| TEXAS INSTRUMENTS INCORPORATED
| Standard Linear and Logic Group
| IBIS Model of SN74CBT3253C
| Dual 1-Of-4 FET Multiplexer/Demultiplexer
| With -2 V Undershoot-Protection
| This file contains package information for the following:
|  SOIC 16-pin (D) package as [Component] CBT3253C_D
|  SSOP 16-pin (DB) package as [Component] CBT3253C_DB
|  SSOP 16-pin (DBQ) package as [Component] CBT3253C_DBQ
|  TSSOP 16-pin (PW) package as [Component] CBT3253C_PW
|  QFN 16-pin (RGY) package as [Component] CBT3253C_RGY
| This device can be powered at the following Vccs:
|  5 volt Vcc
|  4 volt Vcc
| This file provides unique models under the [Model Selector] for each Vcc.
| For operation at a specific Vcc, select the appropriate model after each
| [Model Selector] keyword.
[IBIS Ver]   3.2
[Comment char]  |_char
[File Name]   sn74cbt3253c.ibs
[File Rev]   1.1 | b_die
[Date]   June 25, 2003
[Source]   Data created from TI-SPICE simulations at TI-SLL.
[Notes]   The following is an IBIS list for the CBT3253C.
   Please contact sllibis@ti.com with questions and
   comments concerning SLL IBIS models.
   - Power-clamp data has been deleted since there is no
   power-clamp diode in the device.
   - Non-monotonic data due to FET characteristics.
[Disclaimer] Property of Texas Instruments Incorporated.  Unauthorized
   reproduction and/or distribution is strictly prohibited.
   This product is protected under copyright law.
   Created  2003, (C) Copyright  2003, Texas Instruments
   Incorporated, All Rights Reserved
   UNLESS THERE IS A SIGNED, WRITTEN AGREEMENT TO THE
   CONTRARY, TEXAS INSTRUMENTS (TI) IS PROVIDING THE IBIS
   MODELS  AND WITHOUT ANY WARRANTY, EXPRESSED OR
   IMPLIED.  TI assumes no liability for:
   1) the accuracy of the IBIS models provided to your
   company;
   2) the proper functioning of these IBIS Models in your
   design or for any resulting applications; or
   3) infringement of patents, copyrights or intellectual
   property rights resulting from your use of these IBIS
   models.
   TI provides IBIS Models as a service to our customers.
   You and your company shall not distribute, sell or give
   these models to anyone else without prior written
   permission from TI.
   TI reserves the right to make changes to our products or
   to discontinue any semiconductor product or service
   without notice, and advises our customers to obtain the
   latest version of relevant information to verify, before
   placing orders, that the information being relied on is
   current.
   Please be aware that your receipt and use of the IBIS
   information provided shall serve as acceptance of these
   terms and conditions.  If you do not accept these terms,
   you should return or destroy the IBIS models and any
   other accompanying information immediately.
| Component CBT3253C_D 16-pin SOIC
[Component]   CBT3253C_D
[Manufacturer]   Texas Instruments, Inc.
[Package]
|   typ   min   max
R_pkg   3.900e-02   2.800e-02   4.900e-02
L_pkg   3.453e-09   2.350e-09   4.375e-09
C_pkg   5.210e-13   2.540e-13   7.080e-13
[Pin]   signal_name   model_name   R_pin   L_pin   C_pin
1   1NOE   CBT3253C_IN   4.200e-02   4.336e-09   7.030e-13
2   S1   CBT3253C_IN   4.900e-02   3.778e-09   6.340e-13
3   1B4   CBT3253C_IO   2.800e-02   3.449e-09   5.180e-13
4   1B3   CBT3253C_IO   2.900e-02   2.393e-09   2.540e-13
5   1B2   CBT3253C_IO   2.800e-02   2.350e-09   2.640e-13
6   1B1   CBT3253C_IO   4.800e-02   3.312e-09   4.830e-13
7   1A   CBT3253C_IO   4.300e-02   3.629e-09   6.040e-13
8   GND   GND   4.400e-02   4.375e-09   7.080e-13
9   2A   CBT3253C_IO   4.200e-02   4.336e-09   7.030e-13
10   2B1   CBT3253C_IO   4.900e-02   3.778e-09   6.340e-13
11   2B2   CBT3253C_IO   2.800e-02   3.449e-09   5.180e-13
12   2B3   CBT3253C_IO   2.900e-02   2.393e-09   2.550e-13
13   2B4   CBT3253C_IO   2.800e-02   2.350e-09   2.640e-13
14   S0   CBT3253C_IN   4.800e-02   3.312e-09   4.830e-13
15   2NOE   CBT3253C_IN   4.300e-02   3.629e-09   6.040e-13
16   VCC   POWER   4.400e-02   4.375e-09   7.080e-13
| Component CBT3253C_DB 16-pin SSOP
[Component]   CBT3253C_DB
[Manufacturer]   Texas Instruments, Inc.
[Package]
|   typ   min   max
R_pkg   4.800e-02   4.600e-02   5.000e-02
L_pkg   3.536e-09   3.213e-09   3.798e-09
C_pkg   3.760e-13   3.140e-13   4.400e-13
[Pin]   signal_name   model_name   R_pin   L_pin   C_pin
1   1NOE   CBT3253C_IN   4.800e-02   3.797e-09   3.770e-13
2   S1   CBT3253C_IN   4.600e-02   3.723e-09   4.400e-13
3   1B4   CBT3253C_IO   4.800e-02   3.409e-09   3.720e-13
4   1B3   CBT3253C_IO   4.900e-02   3.213e-09   3.140e-13
5   1B2   CBT3253C_IO   4.900e-02   3.213e-09   3.140e-13
6   1B1   CBT3253C_IO   4.800e-02   3.409e-09   3.720e-13
7   1A   CBT3253C_IO   4.600e-02   3.723e-09   4.400e-13
8   GND   GND   4.800e-02   3.798e-09   3.770e-13
9   2A   CBT3253C_IO   4.800e-02   3.797e-09   3.770e-13
10   2B1   CBT3253C_IO   4.600e-02   3.725e-09   4.400e-13
11   2B2   CBT3253C_IO   4.800e-02   3.409e-09   3.720e-13
12   2B3   CBT3253C_IO   4.900e-02   3.214e-09   3.140e-13
13   2B4   CBT3253C_IO   5.000e-02   3.216e-09   3.140e-13
14   S0   CBT3253C_IN   4.800e-02   3.409e-09   3.720e-13
15   2NOE   CBT3253C_IN   4.700e-02   3.729e-09   4.400e-13
16   VCC   POWER   4.800e-02   3.797e-09   3.770e-13
| Component CBT3253C_DBQ 16-pin SSOP
[Component]   CBT3253C_DBQ
[Manufacturer]   Texas Instruments, Inc.
[Package]
|   typ   min   max
R_pkg   3.800e-02   2.700e-02   5.900e-02
L_pkg   2.353e-09   1.491e-09   4.500e-09
C_pkg   2.100e-13   6.400e-14   5.920e-13
[Pin]   signal_name   model_name   R_pin   L_pin   C_pin
1   1NOE   CBT3253C_IN   5.800e-02   4.450e-09   5.920e-13
2   S1   CBT3253C_IN   4.000e-02   1.930e-09   1.110e-13
3   1B4   CBT3253C_IO   2.800e-02   1.538e-09   7.600e-14
4   1B3   CBT3253C_IO   2.700e-02   1.491e-09   6.400e-14
5   1B2   CBT3253C_IO   2.700e-02   1.491e-09   6.400e-14
6   1B1   CBT3253C_IO   2.700e-02   1.506e-09   7.500e-14
7   1A   CBT3253C_IO   3.300e-02   1.922e-09   1.090e-13
8   GND   GND   5.900e-02   4.500e-09   5.880e-13
9   2A   CBT3253C_IO   5.800e-02   3.695e-09   4.140e-13
10   2B1   CBT3253C_IO   3.400e-02   2.685e-09   2.820e-13
11   2B2   CBT3253C_IO   2.900e-02   1.552e-09   7.700e-14
12   2B3   CBT3253C_IO   2.800e-02   1.506e-09   6.500e-14
13   2B4   CBT3253C_IO   2.700e-02   1.492e-09   6.400e-14
14   S0   CBT3253C_IN   2.800e-02   1.534e-09   7.600e-14
15   2NOE   CBT3253C_IN   4.000e-02   2.703e-09   2.840e-13
16   VCC   POWER   5.600e-02   3.645e-09   4.180e-13
| Component CBT3253C_PW 16-pin TSSOP
[Component]   CBT3253C_PW
[Manufacturer]   Texas Instruments, Inc.
[Package]
|   typ   min   max
R_pkg   4.500e-02   3.800e-02   5.100e-02
L_pkg   2.593e-09   2.447e-09   3.080e-09
C_pkg   2.810e-13   2.430e-13   3.770e-13
[Pin]   signal_name   model_name   R_pin   L_pin   C_pin
1   1NOE   CBT3253C_IN   4.000e-02   3.080e-09   3.770e-13
2   S1   CBT3253C_IN   3.800e-02   2.458e-09   2.810e-13
3   1B4   CBT3253C_IO   5.100e-02   2.512e-09   2.550e-13
4   1B3   CBT3253C_IO   5.100e-02   2.447e-09   2.430e-13
5   1B2   CBT3253C_IO   5.100e-02   2.447e-09   2.430e-13
6   1B1   CBT3253C_IO   5.100e-02   2.512e-09   2.550e-13
7   1A   CBT3253C_IO   3.800e-02   2.458e-09   2.810e-13
8   GND   GND   4.000e-02   3.080e-09   3.770e-13
9   2A   CBT3253C_IO   3.900e-02   2.832e-09   3.160e-13
10   2B1   CBT3253C_IO   3.800e-02   2.460e-09   2.790e-13
11   2B2   CBT3253C_IO   5.100e-02   2.512e-09   2.550e-13
12   2B3   CBT3253C_IO   5.100e-02   2.447e-09   2.430e-13
13   2B4   CBT3253C_IO   5.100e-02   2.447e-09   2.430e-13
14   S0   CBT3253C_IN   5.100e-02   2.512e-09   2.550e-13
15   2NOE   CBT3253C_IN   3.800e-02   2.459e-09   2.790e-13
16   VCC   POWER   3.900e-02   2.832e-09   3.160e-13
| Component CBT3253C_RGY 16-pin QFN
[Component]   CBT3253C_RGY
[Manufacturer]   Texas Instruments, Inc.
[Package]
|   typ   min   max
R_pkg   3.000e-02   2.700e-02   3.800e-02
L_pkg   8.000e-10   7.220e-10   9.400e-10
C_pkg   1.410e-13   1.290e-13   1.550e-13
[Pin]   signal_name   model_name   R_pin   L_pin   C_pin
1   1NOE   CBT3253C_IN   2.700e-02   8.180e-10   1.320e-13
2   S1   CBT3253C_IN   2.700e-02   8.030e-10   1.300e-13
3   1B4   CBT3253C_IO   3.700e-02   9.080e-10   1.500e-13
4   1B3   CBT3253C_IO   2.900e-02   7.220e-10   1.390e-13
5   1B2   CBT3253C_IO   2.900e-02   7.220e-10   1.390e-13
6   1B1   CBT3253C_IO   2.900e-02   7.300e-10   1.400e-13
7   1A   CBT3253C_IO   2.900e-02   7.240e-10   1.390e-13
8   GND   GND   3.100e-02   8.000e-10   1.400e-13
9   2A   CBT3253C_IO   2.700e-02   8.110e-10   1.290e-13
10   2B1   CBT3253C_IO   2.800e-02   7.840e-10   1.310e-13
11   2B2   CBT3253C_IO   3.700e-02   9.150e-10   1.530e-13
12   2B3   CBT3253C_IO   2.900e-02   8.470e-10   1.520e-13
13   2B4   CBT3253C_IO   2.900e-02   7.580e-10   1.430e-13
14   S0   CBT3253C_IN   2.900e-02   7.720e-10   1.440e-13
15   2NOE   CBT3253C_IN   2.900e-02   7.400e-10   1.420e-13
16   VCC   POWER   3.800e-02   9.400e-10   1.550e-13
[Series Switch Groups]
| Function Group States
On  1 /   | 1A->1B1 1noe low, s1 low, s0 low
On  2 /   | 1A->1B2 1noe low, s1 low, s0 high
On  3 /   | 1A->1B3 1noe low, s1 high, s0 low
On  4 /   | 1A->1B4 1noe low, s1 high, s0 high
On  5 /   | 2A->2B1 2noe low, s1 low, s0 low
On  6 /   | 2A->2B2 2noe low, s1 low, s0 high
On  7 /   | 2A->2B3 2noe low, s1 high, s0 low
On  8 /   | 2A->2B4 2noe low, s1 high, s0 high
On  1 5 /   | enable 1 5
On  2 6 /   | enable 2 6
On  3 7 /   | enable 3 7
On  4 8 /   | enable 4 8
Off  1 2 3 4 /   | disable 1 2 3 4, 1noe high
Off  5 6 7 8 /   | disable 5 6 7 8, 2noe high
Off 1 2 3 4 5 6 7 8 /  | disable all, 1noe high, 2noe high
[Series Pin Mapping]   pin_2   model_name   function_table_group
7   6   CBT3253C_IO_50_S   1
| 7   6   CBT3253C_IO_40_S   1
7   5   CBT3253C_IO_50_S   2
| 7   5   CBT3253C_IO_40_S   2
7   4   CBT3253C_IO_50_S   3
| 7   4   CBT3253C_IO_40_S   3
7   3   CBT3253C_IO_50_S   4
| 7   3   CBT3253C_IO_40_S   4
9   10   CBT3253C_IO_50_S   5
| 9   10   CBT3253C_IO_40_S   5
9   11   CBT3253C_IO_50_S   6
| 9   11   CBT3253C_IO_40_S   6
9   12   CBT3253C_IO_50_S   7
| 9   12   CBT3253C_IO_40_S   7
9   13   CBT3253C_IO_50_S   8
| 9   13   CBT3253C_IO_40_S   8
| Model CBT3253C_IN
[Model Selector]   CBT3253C_IN
CBT3253C_IN_50   5 volt Vcc
CBT3253C_IN_40   4 volt Vcc
| Model CBT3253C_IO
[Model Selector]   CBT3253C_IO
CBT3253C_IO_50   5 volt Vcc
CBT3253C_IO_40   4 volt Vcc
| Model CBT3253C_IO_S
[Model Selector]   CBT3253C_IO_S
CBT3253C_IO_50_S   5 volt Vcc
CBT3253C_IO_40_S   4 volt Vcc
[Model]   CBT3253C_IO_50_S
Model_type  Series_switch
| variable   typ   min   max
C_comp   0   0   0
[Temperature Range]   40   100   -40
| Ambient temperature   25   85   -40
[Voltage range]   5   4.5   5.5
[On]
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[Off]
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[Model]   CBT3253C_IO_40_S
Model_type  Series_switch
| variable   typ   min   max
C_comp   0   0   0
[Temperature Range]   40   100   -40
| Ambient temperature   25   85   -40
[Voltage range]   4   4   4
[On]
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[Off]
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| Models and submodels in the file (6): CBT3253C_IN_50 (Input), CBT3253C_IN_40 (Input), CBT3253C_IO_50_S (Series_switch), CBT3253C_IO_50 (Terminator), CBT3253C_IO_40_S (Series_switch), CBT3253C_IO_40 (Terminator)
